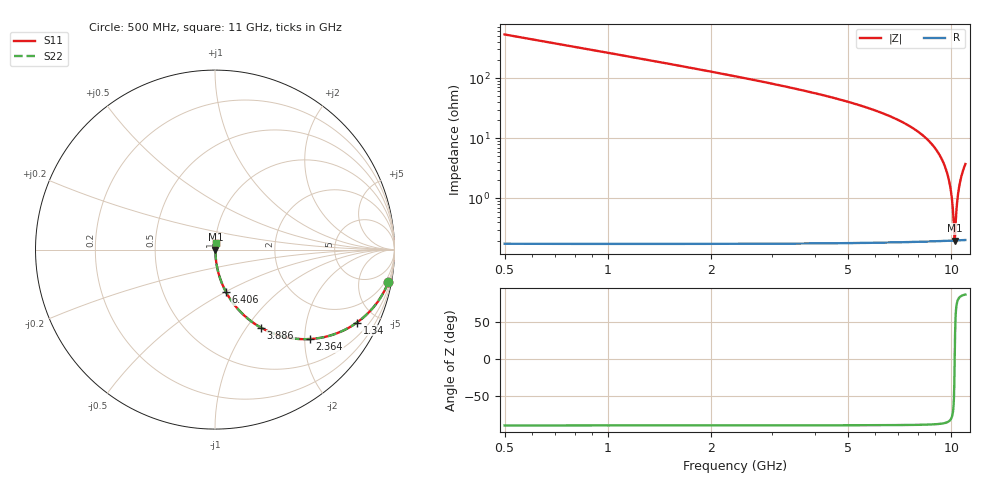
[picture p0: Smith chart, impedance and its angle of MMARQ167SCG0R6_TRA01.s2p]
! MMARQ167SCG0R6_TRA01  S-PARAMETER MODEL  ( General Type )
! Model Generated by TAIYO YUDEN Corporation (http://www.ty-top.com)
! Version 1.0
! TAIYO YUDEN Control No. 160201
! Copyright(c) 2016 TAIYO YUDEN CO.,LTD. All Rights Reserved.
! Product Description (link to TY-COMPAS)
! https://ds.yuden.co.jp/TYCOMPAS/or/detail?pn=MMARQ167SCG0R6BTRA01&u=M
! Products Name : Multilayer Ceramic Capacitors
! Characteristics :
!  Capacitance : 0.6 pF , Rated Voltage : 250V , TCC : CG / C0G
!  Case Size : 1.6 x 0.8 / 0.063 x 0.031 [mm/inch] , Thickness : 0.7 / 0.028 [mm/inch]
!  (Conditions: Temperature = 25 degC , DC Bias Current/Voltage = 0A / 0V)
! External Node Assignments :
!  1  o---| |---o  2
! GND o---------o GND
! Frequency Range : 500MHz  -  11000MHz  [ 401 STEP ]
# MHz S RI R 50
! Freq[MHz].  S11 Real  S11 Imag  S21 Real  S21 Imag  S12 Real  S12 Imag  S22 Real  S22 Imag
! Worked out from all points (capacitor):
!   401 points, 500 MHz to 11 GHz, reference 50 ohm
!   read as one part in series: C = 600 fF near 552.5 MHz
!   lowest |Z| = 200 mohm at 10.24 GHz (marker M1)
!   series resonance near 10.24 GHz, so ESL is about 400 pH
!   S11 on the Smith chart (normalised r, x): 500 MHz: 1, -11; 1.34 GHz: 1.00, -3.89; 2.364 GHz: 1.00, -2.13; 3.886 GHz: 1.00, -1.17; 6.406 GHz: 1.00, -0.50; 11 GHz: 1.00, +0.07
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500  0.9655 -0.1824  0.0345 0.1824  0.0345 0.1824  0.9655 -0.1824
893.75  0.8965 -0.3043  0.1035 0.3043  0.1035 0.3043  0.8965 -0.3043
1340  0.7909 -0.4062  0.2091 0.4062  0.2091 0.4062  0.7909 -0.4062
2258.75  0.5552 -0.4962  0.4448 0.4962  0.4448 0.4962  0.5552 -0.4962
2363.75  0.5302 -0.4983  0.4698 0.4983  0.4698 0.4983  0.5302 -0.4983
3886.25  0.2552 -0.4344  0.7448 0.4344  0.7448 0.4344  0.2552 -0.4344
4017.5  0.2386 -0.4246  0.7614 0.4246  0.7614 0.4246  0.2386 -0.4246
5750  0.0921 -0.2863  0.9079 0.2863  0.9079 0.2863  0.0921 -0.2863
6406.25  0.0612 -0.2361  0.9388 0.2361  0.9388 0.2361  0.0612 -0.2361
7508.75  0.0277 -0.1585  0.9723 0.1585  0.9723 0.1585  0.0277 -0.1585
8532.5  0.0108 -0.0938  0.9892 0.0938  0.9892 0.0938  0.0108 -0.0938
9267.5  0.00461 -0.0514  0.9954 0.0514  0.9954 0.0514  0.00461 -0.0514
9635  0.00296 -0.0314  0.997 0.0314  0.997 0.0314  0.00296 -0.0314
9897.5  0.00229 -0.0175  0.9977 0.0175  0.9977 0.0175  0.00229 -0.0175
10055  0.00208 -0.00934  0.9979 0.00934  0.9979 0.00934  0.00208 -0.00934
10186.25  0.002 -0.00264  0.998 0.00264  0.998 0.00264  0.002 -0.00264
10238.75  0.002 9.76e-06  0.998 -9.76e-06  0.998 -9.76e-06  0.002 9.76e-06
10291.25  0.00201 0.00265  0.998 -0.00265  0.998 -0.00265  0.00201 0.00265
10396.25  0.00207 0.00789  0.9979 -0.00789  0.9979 -0.00789  0.00207 0.00789
10527.5  0.00222 0.0144  0.9978 -0.0144  0.9978 -0.0144  0.00222 0.0144
10737.5  0.00263 0.0246  0.9974 -0.0246  0.9974 -0.0246  0.00263 0.0246
11000  0.00341 0.037  0.9966 -0.037  0.9966 -0.037  0.00341 0.037
